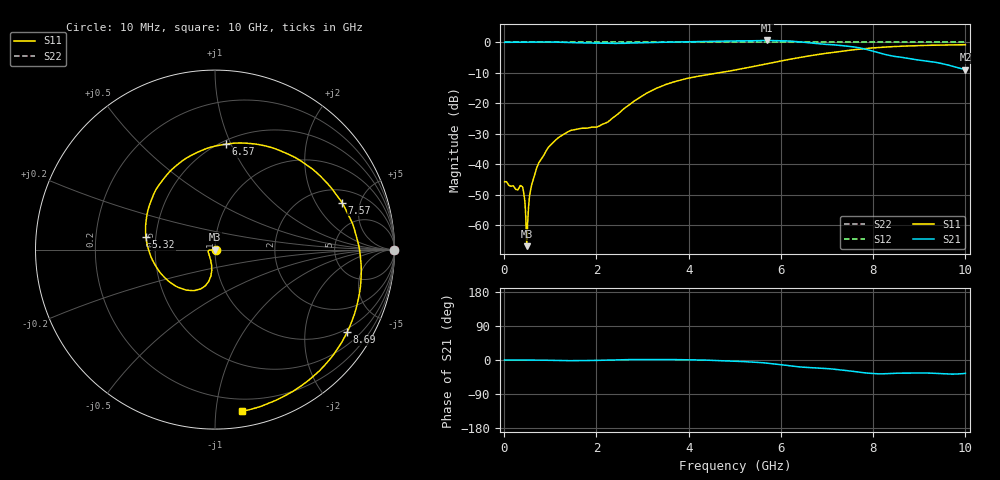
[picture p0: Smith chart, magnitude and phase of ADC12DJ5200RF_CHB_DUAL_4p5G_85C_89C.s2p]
! Texas Instruments, Inc.
! ADC12DJ5200RF - CH B S-Parameters (Dual Ch Mode, Fs = 4.5 GSPS, 85 degC case, 89 degC juntion)
! Port 1 represents the 100-ohm differenal input, Port 2 the digital output
! freq  dbS11  angS11  dbS21 angS21 dbS12 angS12 dbS22 angS22
# HZ S DB R 100
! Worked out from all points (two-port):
!   1000 points, 10 MHz to 10 GHz, reference 100 ohm
!   highest |S21| = 0.61 dB at 5.69 GHz (marker M1); lowest = -9.0 dB at 10 GHz (marker M2)
!   |S21| within 3 dB of the highest: start of sweep to 7.87 GHz
!   lowest |S11| = -66.8 dB at 490 MHz (marker M3), VSWR 1.00, Z = 100 + j0.0909 ohm
!   |S11| at or under -10 dB: start of sweep to 4.655 GHz
!   |S22| runs from 0.0 to 0.0 dB; largest |S21 - S12| = 0.74
!   S11 on the Smith chart (normalised r, x): 10 MHz: 1.01, -0.00; 5.32 GHz: 0.44, +0.07; 6.57 GHz: 0.53, +0.96; 7.57 GHz: 2.79, +3.39; 8.69 GHz: 0.87, -3.26; 10 GHz: 0.11, -1.18
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1e7  -45.69 -2.8  0.00 0.0  0.00 0.0  0.00 0.0
3.8e8  -47.17 -16.4  0.04 -0.0  0.00 0.0  0.00 0.0
4.9e8  -66.84 93.5  0.05 -0.1  0.00 0.0  0.00 0.0
5.2e8  -56.15 -177.4  0.06 -0.1  0.00 0.0  0.00 0.0
5.8e8  -47.93 -158.5  0.07 -0.2  0.00 0.0  0.00 0.0
6.5e8  -44.16 -162.0  0.07 -0.3  0.00 0.0  0.00 0.0
9.2e8  -35.36 -172.3  0.11 -0.7  0.00 0.0  0.00 0.0
1.25e9  -30.53 -174.5  0.02 -1.5  0.00 0.0  0.00 0.0
1.68e9  -28.19 -167.0  -0.17 -1.5  0.00 0.0  0.00 0.0
2.22e9  -26.31 -127.8  -0.30 -0.7  0.00 0.0  0.00 0.0
3.34e9  -14.84 -101.2  -0.00 1.4  0.00 0.0  0.00 0.0
4.23e9  -11.08 -126.9  0.26 0.2  0.00 0.0  0.00 0.0
5.01e9  -9.07 -169.7  0.45 -3.3  0.00 0.0  0.00 0.0
5.32e9  -8.17 169.9  0.49 -4.9  0.00 0.0  0.00 0.0
5.69e9  -7.06 144.7  0.61 -8.3  0.00 0.0  0.00 0.0
6.57e9  -4.57 84.1  -0.09 -19.6  0.00 0.0  0.00 0.0
6.67e9  -4.31 77.3  -0.26 -20.5  0.00 0.0  0.00 0.0
7.09e9  -3.36 49.3  -0.74 -23.5  0.00 0.0  0.00 0.0
7.57e9  -2.45 20.4  -1.49 -30.0  0.00 0.0  0.00 0.0
8.34e9  -1.48 -18.1  -4.25 -35.9  0.00 0.0  0.00 0.0
8.69e9  -1.23 -32.1  -5.12 -34.8  0.00 0.0  0.00 0.0
1e10  -0.78 -80.5  -8.96 -35.3  0.00 0.0  0.00 0.0
